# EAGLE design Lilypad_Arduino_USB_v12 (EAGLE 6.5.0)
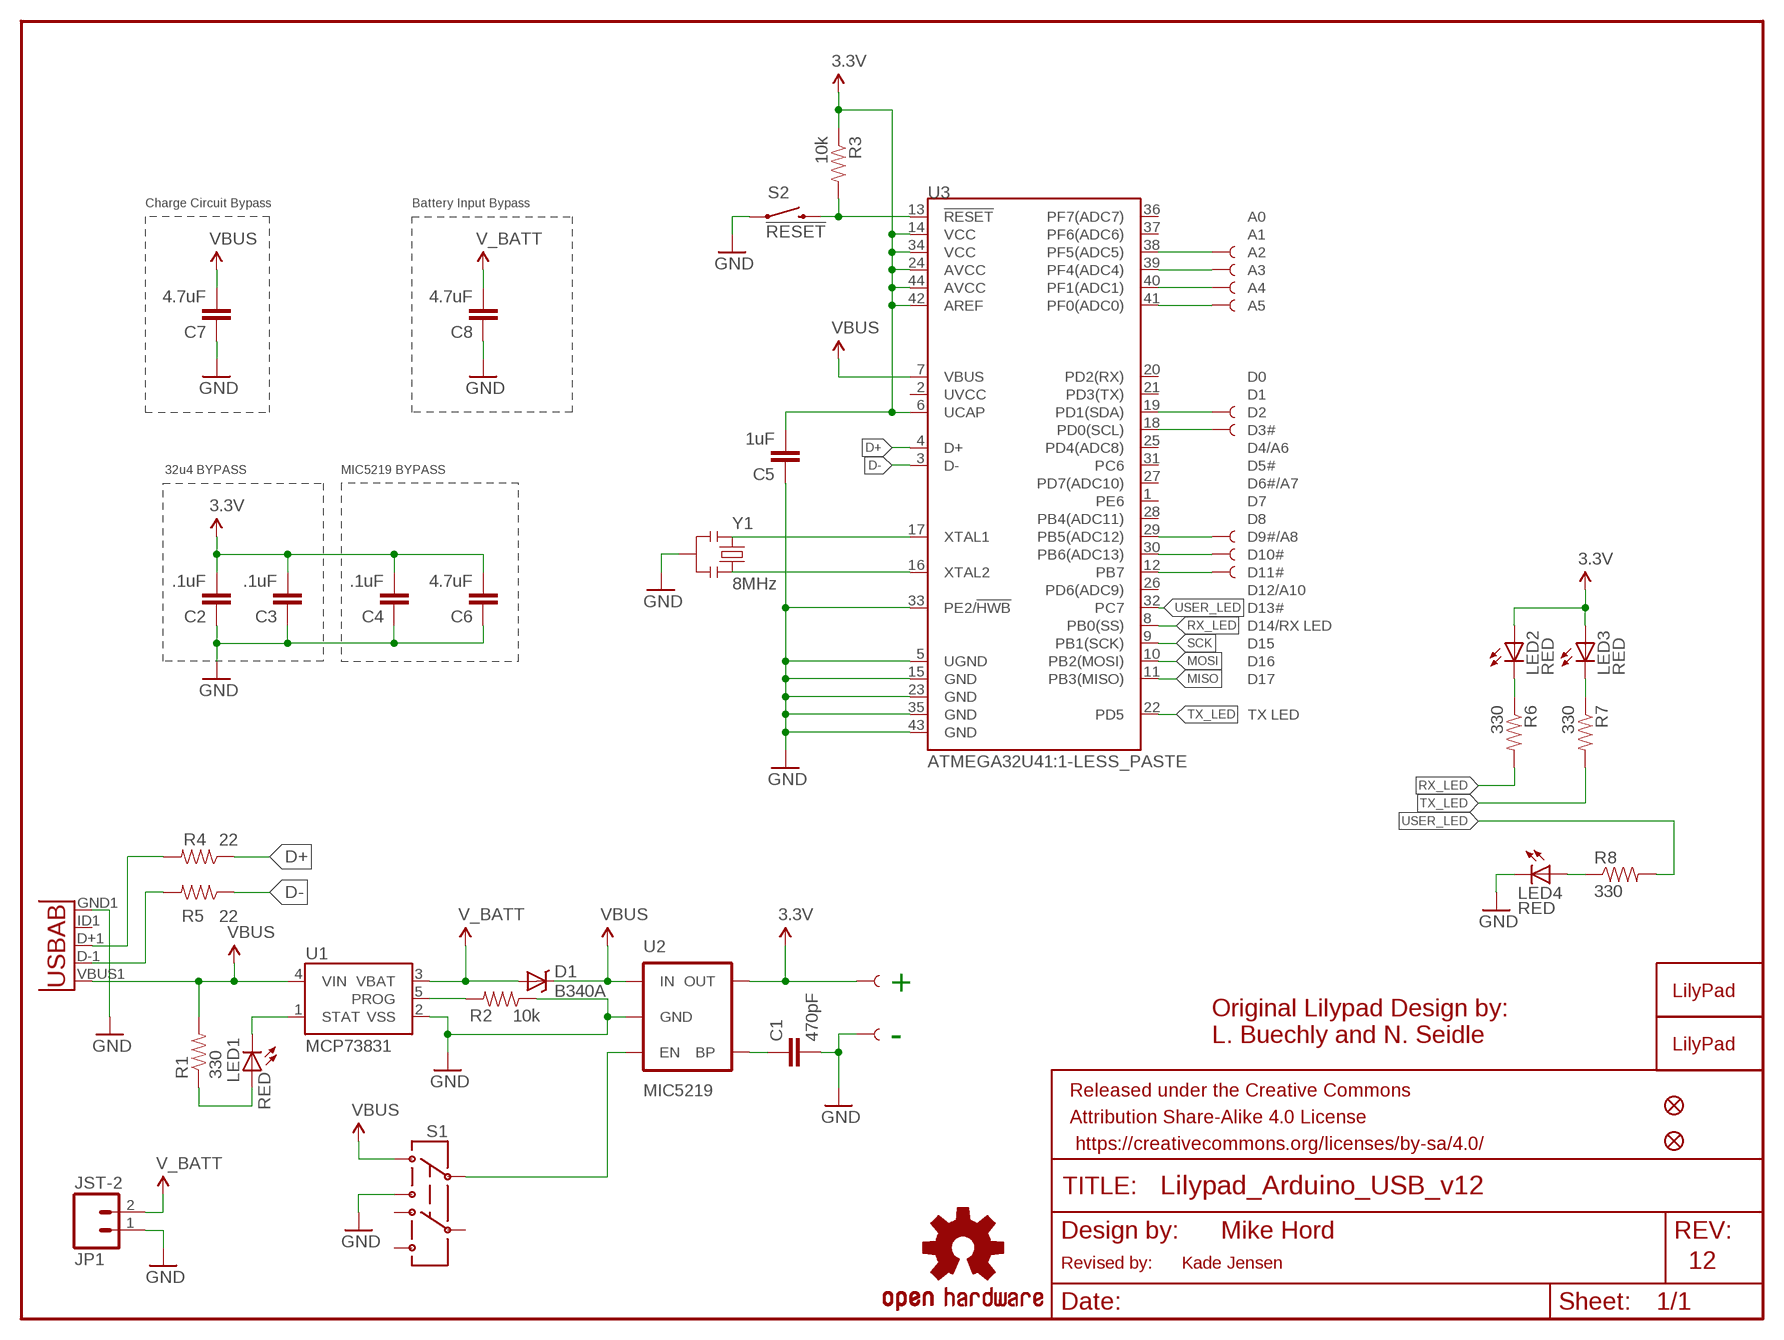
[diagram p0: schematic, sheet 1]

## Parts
+  SEWTAP9  [PETAL-LONG-1-2SIDE]
-  SEWTAP9  [PETAL-LONG-1-2SIDE]
A2  SEWTAP9  [PETAL-LONG-1-2SIDE]
A3  SEWTAP9  [PETAL-LONG-1-2SIDE]
A4  SEWTAP9  [PETAL-LONG-1-2SIDE]
A5  SEWTAP9  [PETAL-LONG-1-2SIDE]
C1  470pF  CAP0603-CAP  [0603-CAP]
C2  .1uF  CAP0603-CAP  [0603-CAP]
C3  .1uF  CAP0603-CAP  [0603-CAP]
C4  .1uF  CAP0603-CAP  [0603-CAP]
C5  1uF  CAP0603-CAP  [0603-CAP]
C6  4.7uF  CAP0603-CAP  [0603-CAP]
C7  4.7uF  CAP1206  [1206]
C8  4.7uF  CAP1206  [1206]
D1  B340A  DIODE-SCHOTTKY-B340A  [SMA-DIODE]
D5  SEWTAP9  [PETAL-LONG-1-2SIDE]
D6  SEWTAP9  [PETAL-LONG-1-2SIDE]
D9  SEWTAP9  [PETAL-LONG-1-2SIDE]
D10  SEWTAP9  [PETAL-LONG-1-2SIDE]
D11  SEWTAP9  [PETAL-LONG-1-2SIDE]
FRAME1  FRAME-LETTER  [CREATIVE_COMMONS]
JP1  JST-2  M02-JST-2MM-SMT  [JST-2-SMD]
JP2  FIDUCIAL1X2  [FIDUCIAL-1X2]
JP3  FIDUCIAL1X2  [FIDUCIAL-1X2]
LED1  RED  LED0603  [LED-0603]
LED2  RED  LED0603  [LED-0603]
LED3  RED  LED0603  [LED-0603]
LED4  RED  LED0603  [LED-0603]
R1  330  RESISTOR0603-RES  [0603-RES]
R2  10k  RESISTOR0603-RES  [0603-RES]
R3  10k  RESISTOR0603-RES  [0603-RES]
R4  22  RESISTOR0603-RES  [0603-RES]
R5  22  RESISTOR0603-RES  [0603-RES]
R6  330  RESISTOR0603-RES  [0603-RES]
R7  330  RESISTOR0603-RES  [0603-RES]
R8  330  RESISTOR0603-RES  [0603-RES]
S1  SWITCH-DPDTAYZ0202  [AYZ0202]
S2  !RESET  SWITCH-MOMENTARY-2SMD  [TACTILE_SWITCH_SMD]
U1  MCP73831  [SOT23-5]
U2  MIC5219  V_REG_MIC52193.3V  [SOT23-5]
U3  ATMEGA32U41:1-LESS_PASTE  [QFN-44-NOPAD_1:1-LESS_PASTE]
U5  USB-ABCONN-11794  [USB-AB-MICRO-SMD_V03]
U$1  LOGO-LPLPA  [LOGO-LPA]
U$5  OSHW-LOGOM  [OSHW-LOGO-M]
U$13  LOGO-LPLP  [LOGO-LILYPAD]
Y1  8MHz  RESONATOR8MHZ  [RESONATOR-SMD]

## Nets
3.3V: +.1 C2.2 C3.2 C4.2 C5.2 C6.2 LED2.A LED3.A R3.1 U2.5(OUT) U3.6(UCAP) U3.14(VCC) U3.24(AVCC) U3.34(VCC) U3.42(AREF) U3.44(AVCC)
5V: C7.2 D1.C R1.2 S1.1 U1.4(VIN) U2.1(IN) U3.7(VBUS) U5.VBUS1(VBUS) ; supply symbol labelled VBUS
D+: R4.1 U3.4(D+)
D-: R5.1 U3.3(D-)
GND: -.1 C1.2 C2.1 C3.1 C4.1 C5.1 C6.1 C7.1 C8.1 JP1.1 LED4.C R2.1 S1.3 S2.1 U1.2(VSS) U2.2(GND) U3.5(UGND) U3.15(GND) U3.23(GND) U3.33(PE2/!HWB) U3.35(GND) U3.43(GND) U5.GND1(GND) Y1.2
MISO: U3.11(PB3(MISO))
MOSI: U3.10(PB2(MOSI))
N$1: LED2.C R6.1
N$2: S1.2 U2.3(EN)
N$3: LED1.A R1.1
N$4: LED1.C U1.1(STAT)
N$5: U3.17(XTAL1) Y1.1
N$6: R2.2 U1.5(PROG)
N$7: U3.16(XTAL2) Y1.3
N$8: C1.1 U2.4(BP)
N$9: D11.1 U3.12(PB7)
N$10: D10.1 U3.30(PB6(ADC13))
N$11: D9.1 U3.29(PB5(ADC12))
N$12: D5.1 U3.19(PD1(SDA))
N$13: D6.1 U3.18(PD0(SCL))
N$14: A5.1 U3.41(PF0(ADC0))
N$15: A4.1 U3.40(PF1(ADC1))
N$16: A3.1 U3.39(PF4(ADC4))
N$17: A2.1 U3.38(PF5(ADC5))
N$18: LED4.A R8.1
N$19: R5.2 U5.D-1(D-)
N$20: R4.2 U5.D+1(D+)
N$21: LED3.C R7.1
RESET: R3.2 S2.3 U3.13(!RESET)
RX_LED: R6.2 U3.8(PB0(SS))
SCK: U3.9(PB1(SCK))
TX_LED: R7.2 U3.22(PD5)
USER_LED: R8.2 U3.32(PC7)
V_BATT: C8.2 D1.A JP1.2 U1.3(VBAT)
Unconnected: S1.4 S1.5 S1.6 U3.1(PE6) U3.2(UVCC) U3.20(PD2(RX)) U3.21(PD3(TX)) U3.25(PD4(ADC8)) U3.26(PD6(ADC9)) U3.27(PD7(ADC10)) U3.28(PB4(ADC11)) U3.31(PC6) U3.36(PF7(ADC7)) U3.37(PF6(ADC6)) U5.ID1(USBID)

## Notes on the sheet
- Charge Circuit Bypass | Battery Input Bypass
- 32u4 BYPASS | MIC5219 BYPASS
- +
- Original Lilypad Design by:
- - | L. Buechly and N. Seidle
- Mike Hord
- Revised by: | Kade Jensen | 12

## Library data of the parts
+ - A2-A5 D5 D6 D9-D11 = LilyPad-Wearables:SEWTAP; NO_PART: 1
C1 = SparkFun-Passives:CAP: Capacitor; PROD_ID: CAP-07884
C2-C4 = SparkFun-Passives:CAP: Capacitor; PROD_ID: CAP-00810
C5 = SparkFun-Passives:CAP: Capacitor; PROD_ID: CAP-00868
C6 = SparkFun-Passives:CAP: Capacitor; PROD_ID: CAP-08280
C7 C8 = SparkFun-Passives:CAP: Capacitor; PROD_ID: CAP-10300
D1 = SparkFun-DiscreteSemi:DIODE-SCHOTTKY: Schottky diodes in SFE's production catalog; PROD_ID: DIO-09886
FRAME1 = SparkFun-Aesthetics:FRAME-LETTER: Schematic Frame
JP1 = SparkFun-Connectors:M02: Standard 2-pin 0.1" header. Use with; PROD_ID: CONN-08352
JP2 JP3 = SparkFun:FIDUCIAL: Fiducial Alignment Points
LED1-LED4 = SparkFun-LED:LED: LEDs; PROD_ID: DIO-00819
R1 R7 R8 = SparkFun-Passives:RESISTOR: Resistor; PROD_ID: RES-00818
R2 R3 = SparkFun-Resistors:RESISTOR: Resistor; PROD_ID: RES-00824
R4 R5 = SparkFun-Resistors:RESISTOR: Resistor; PROD_ID: RES-08698
R6 = SparkFun-Resistors:RESISTOR: Resistor; PROD_ID: RES-00818
S1 = SparkFun-Electromechanical:SWITCH-DPDT: DPDT Version of the COM-00597; PROD_ID: SWCH-08179; VALUE: DPDT
S2 = SparkFun-Electromechanical:SWITCH-MOMENTARY-2: Various NO switches- pushbuttons, reed, etc; PROD_ID: SWCH-08247
U1 = SparkFun-PowerIC:MCP73831: Miniature single cell, fully integrated Li-Ion, Li-polymer charge management controller http://ww1.microchip.com/downloads/en/DeviceDoc/21984a.pdf IC-09995; PROD_ID: IC-09995
U2 = SparkFun-PowerIC:V_REG_MIC5219: V_REG MIC5219 Standard 3.3V and 5V 500mA LDO voltage regulator in SOT-23 layout. Micrel part MIC5219. BP (by-pass) pin is used to lower output noise with 470pF cap, may be left open.; PROD_ID: VREG-09872; VALUE: MIC5219 3.3V
U3 = Testing:ATMEGA32U4: Atmel 44-pin 8-bit Microcontroller with 32KBytes of ISP Flash and USB Controller; PROD_ID: IC-10828
U5 = SparkFun-Connectors:USB-AB: This is a USB AB connector that is compatible with USB OTG. i.e. this connector can serve as a host or device; PROD_ID: CONN-11794
U$1 = LilyPad-Wearables:LOGO-LP
U$5 = SparkFun:OSHW-LOGO: Open Source Hardware Logo This logo indicates the piece of hardware it is found on incorporates a OSHW license and/or adheres to the definition of open source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
U$13 = LilyPad-Wearables:LOGO-LP; NO_PART: 1
Y1 = SparkFun-FreqCtrl:RESONATOR: Resonator Small SMD resonator. Used, eg, on the Arduino Pro/ Pro Mini boards. 8MHz- XTAL-08895 16MHz- XTAL-08900; PROD_ID: XTAL-08895; VALUE: 8MHZ

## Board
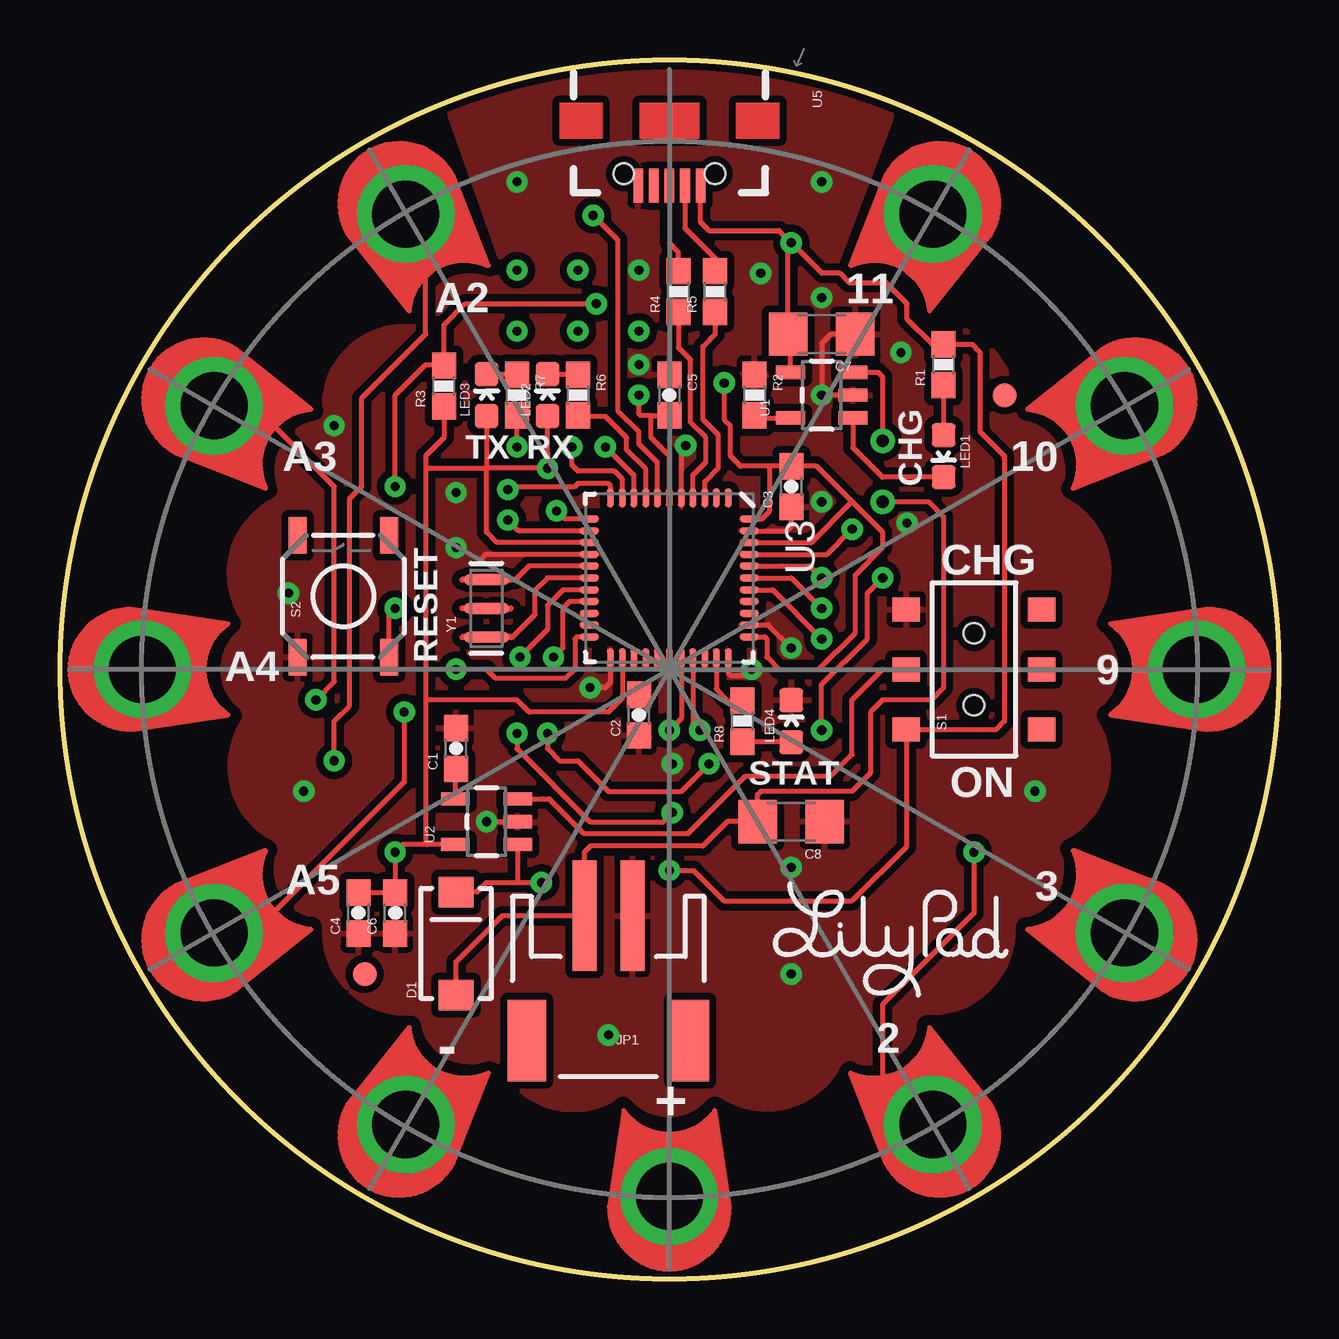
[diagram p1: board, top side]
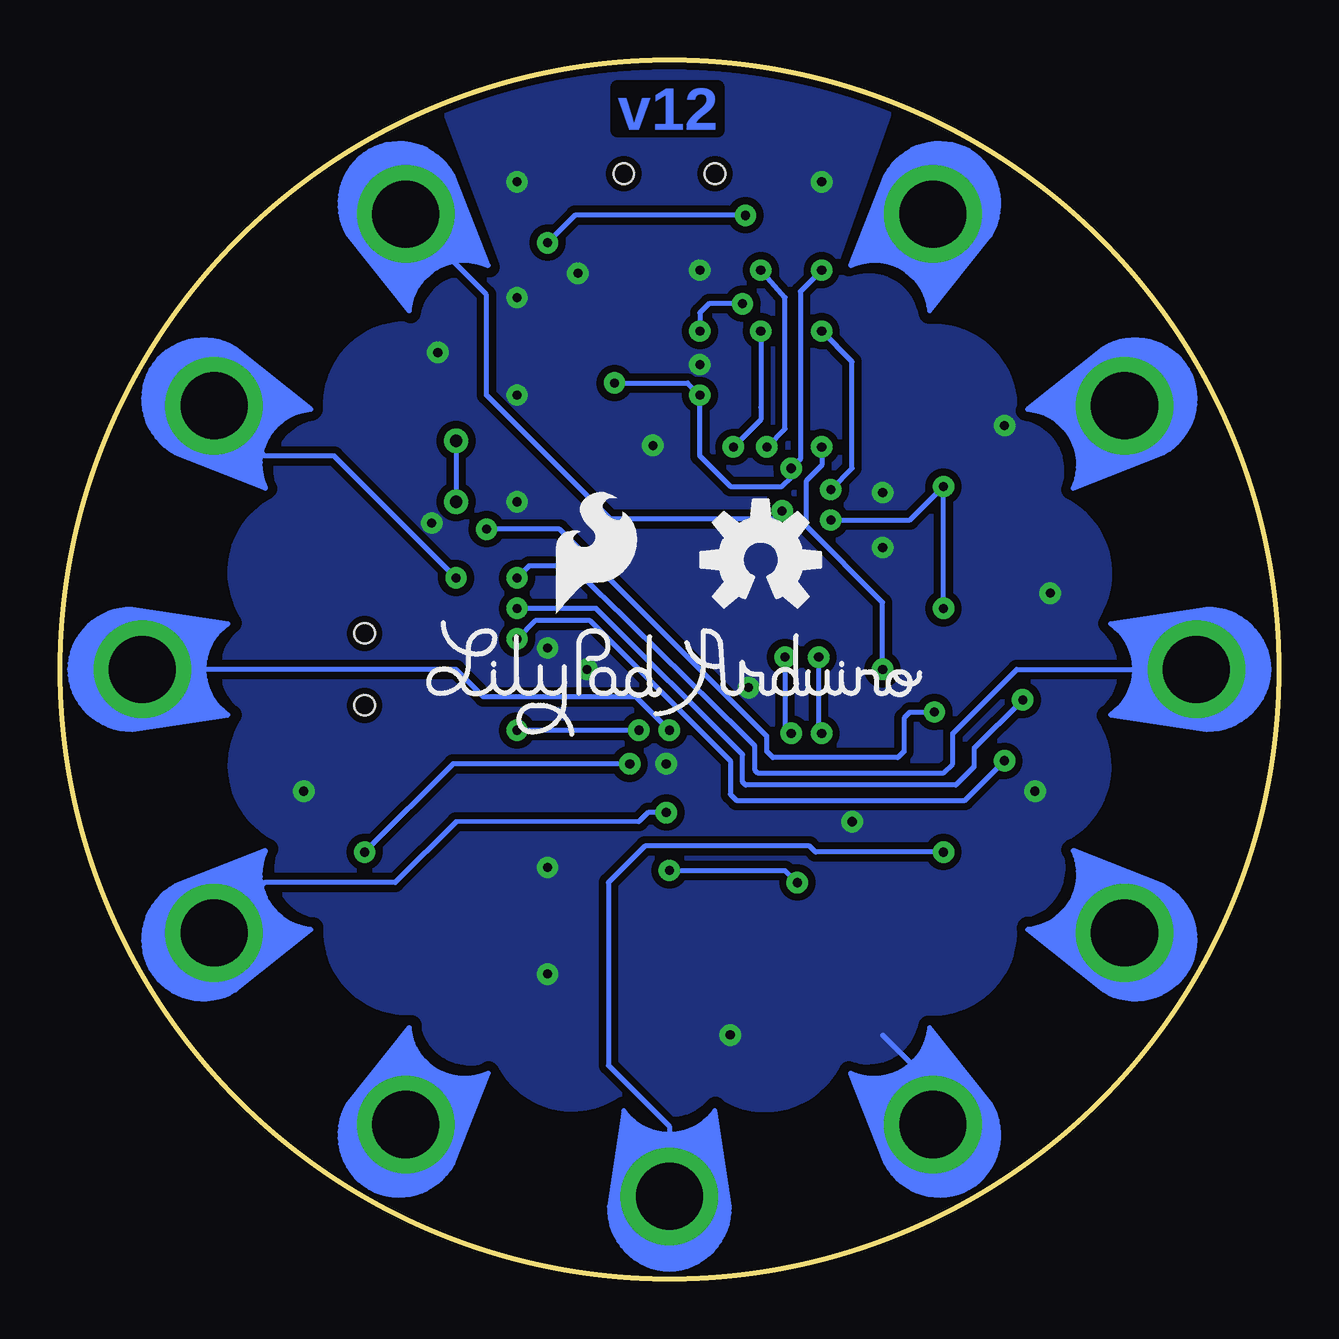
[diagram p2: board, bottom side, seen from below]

Size 50.8 x 50.8 mm. Coordinates in mm from the lower left corner, seen from the top.
Outline: circle at 25.4,25.4 radius 25.4
Copper layers (1*16): Top 0.035mm / dielectric 1.5mm / Bottom 0.035mm
Design rules "SparkFun-2-layer": minimum track width 7mil, minimum drill 15mil, track to track 8mil, track to pad 8mil, pad to pad 8mil, via to via 8mil, smd to smd 8mil, copper to edge 8mil, drill to drill 8mil, minimum pad ring 12mil, minimum via ring 10mil, stop-mask expansion 4mil, vias tented up to drill 20mil, thermal gap 10mil
tRestrict: area 2.1,32.9 to 10.5,40.7; area 40.3,10.1 to 48.7,17.9; area 0.3,22.4 to 7.1,28.6; area 43.7,22.2 to 50.5,28.4; area 32.9,2 to 40.6,10.5; area 40.3,32.9 to 48.8,40.6; area 2,10.2 to 10.5,17.9; area 10.2,40.3 to 17.9,48.8; area 32.9,40.3 to 40.7,48.7; area 10.1,2.1 to 17.9,10.5; area 0.3,27.3 to 8.6,35.3; area 5.2,36.2 to 14.6,45.6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
bRestrict: area 0.3,22.4 to 7.1,28.6; area 43.7,22.2 to 50.5,28.4; area 32.9,2 to 40.6,10.5; area 40.3,32.9 to 48.8,40.6; area 2,10.2 to 10.5,17.9; area 10.2,40.3 to 17.9,48.8; area 32.9,40.3 to 40.7,48.7; area 10.1,2.1 to 17.9,10.5; area 0.3,27.3 to 8.6,35.3; area 5.2,36.2 to 14.6,45.6; area 42.2,27.3 to 50.5,35.3; area 36.2,36.2 to 45.6,45.6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

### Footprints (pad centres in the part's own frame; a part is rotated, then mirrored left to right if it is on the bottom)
PETAL-LONG-1-2SIDE = drill 2.794 pad 4.064: 1 0.03,0
0603-CAP = smd 1.1 x 1: 1 -0.85,0; 2 0.85,0
1206 = smd 1.6 x 1.8: 1 -1.4,0; 2 1.4,0
SMA-DIODE = smd 1.27 x 1.47: A -2.15,0; C 2.15,0
JST-2-SMD = smd 1 x 4.6: 1 -1,-3.7; 2 1,-3.7 | smd 1.6 x 3.4: NC1 -3.4,1.5; NC2 3.4,1.5
FIDUCIAL-1X2 = smd 1 x 1: 1 0,0
LED-0603 = smd 1 x 1: A 0,-0.877; C 0,0.877
0603-RES = smd 1.1 x 1: 1 -0.85,0; 2 0.85,0
AYZ0202 = smd 1 x 1.15: 1 -2.5,2.825; 2 0,2.825; 3 2.5,2.825; 4 -2.5,-2.825; 5 0,-2.825; 6 2.5,-2.825 | hole 0.85: 1.5,0; -1.5,0
TACTILE_SWITCH_SMD = smd 1.524 x 0.762: 1 -2.54,1.905; 2 2.54,1.905; 3 -2.54,-1.905; 4 2.54,-1.905
SOT23-5 = smd 0.55 x 1.2: 1 -0.95,-1.3; 2 0,-1.3; 3 0.95,-1.3; 4 0.95,1.3; 5 -0.95,1.3
QFN-44-NOPAD_1:1-LESS_PASTE = smd 0.8 x 0.3: 1 -3.337,2.458; 2 -3.337,1.958; 3 -3.337,1.479; 4 -3.337,0.979; 5 -3.337,0.5; 6 -3.337,0; 7 -3.337,-0.5; 8 -3.337,-0.979; 9 -3.337,-1.479; 10 -3.337,-1.958; 11 -3.337,-2.458; 23 3.337,-2.458; 24 3.337,-1.958; 25 3.337,-1.479; 26 3.337,-0.979; 27 3.337,-0.5; 28 3.337,0; 29 3.337,0.5; 30 3.337,0.979; 31 3.337,1.479; 32 3.337,1.958; 33 3.337,2.458 | smd 0.3 x 0.8: 12 -2.458,-3.337; 13 -1.958,-3.337; 14 -1.479,-3.337; 15 -0.979,-3.337; 16 -0.5,-3.337; 17 0,-3.337; 18 0.5,-3.337; 19 0.979,-3.337; 20 1.479,-3.337; 21 1.958,-3.337; 22 2.458,-3.337; 34 2.458,3.337; 35 1.958,3.337; 36 1.479,3.337; 37 0.979,3.337; 38 0.5,3.337; 39 0,3.337; 40 -0.5,3.337; 41 -0.979,3.337; 42 -1.479,3.337; 43 -1.958,3.337; 44 -2.458,3.337
USB-AB-MICRO-SMD_V03 = smd 1.4 x 0.4: D+1 2.7,0; D-1 2.7,0.65; GND1 2.7,-1.3; ID1 2.7,-0.65; VBUS1 2.7,1.3 | hole 0.85: 2.2,1.9; 2.2,-1.9
RESONATOR-SMD = smd 0.45 x 1.905: 1 -1.2,0; 2 0,0; 3 1.2,0

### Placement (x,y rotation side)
+  25.4,3.4 90 top
-  14.4,6.4 60 top
A2  14.4,44.4 300 top
A3  6.4,36.4 330 top
A4  3.4,25.4 0 top
A5  6.4,14.4 30 top
C1  16.51,22.1 90 top
C2  24.13,23.5 90 top
C3  30.48,33.02 90 top
C4  12.45,15.24 90 top
C5  25.4,36.83 270 top
C6  13.97,15.24 90 top
C7  31.75,39.37 180 top
C8  30.48,19.05 180 top
D1  16.51,13.97 90 top
D5  36.4,6.4 120 top
D6  44.4,14.4 150 top
D9  47.4,25.4 180 top
D10  44.4,36.4 210 top
D11  36.4,44.4 240 top
FRAME1  not placed on the board
JP1  22.86,11.43 180 top
JP2  12.7,12.7 0 top
JP3  39.37,36.83 0 top
LED1  36.83,34.29 180 top
LED2  20.32,36.83 0 top
LED3  17.78,36.83 0 top
LED4  30.48,23.24 0 top
R1  36.83,38.1 90 top
R2  28.96,36.83 270 top
R3  16,37.21 90 top
R4  25.78,41.15 90 top
R5  27.3,41.15 90 top
R6  21.59,36.83 270 top
R7  19.05,36.83 270 top
R8  28.45,23.24 90 top
S1  38.1,25.4 90 top
S2  11.81,28.45 90 top
U1  31.75,36.83 90 top
U2  17.78,19.05 90 top
U3  25.4,29.21 270 top
U5  25.4,48.26 270 top
U$1  25.4,25.4 0 bottom
U$5  21.59,29.97 0 bottom
U$7  [SFE_LOGO_FLAME_.2]  30.48,27.43 0 bottom
U$13  34.67,14.48 0 top
Y1  17.78,27.94 90 top

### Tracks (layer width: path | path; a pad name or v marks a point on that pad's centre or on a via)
3.3V  (via drill 0.38)
  Top 0.203: 16.19,18.1 U2.5 15.3,18.1 | LED2.A 20.32,34.42 v20.32,33.78 17.78,33.78 | 15.3,18.1 15.24,18.16 15.24,24.13 | 15.3,18.1 14.29,18.1 v13.97,17.78 C6.2 C4.2 | R3.1 16,35.05 15.24,34.29 15.24,33.78 | 29.59,33.87 C3.2 31.53,33.87 33.02,32.38 | U3.44 29.25,31.67 29.59,32 29.59,33.87 | 15.24,24.13 19.05,24.13 19.56,23.62 22.86,23.62 23.44,24.2 23.44,24.34 | U3.24 23.44,24.34 | C2.2 23.44,24.34 | 24.64,35.98 24.22,35.98 24.13,36.07 v24.13,36.83 | U3.6 25.4,34.29 24.64,35.05 24.64,35.98 | 24.64,35.98 C5.2 | v27.69,37.34 27.69,35.81 27.94,35.56 27.94,34.29 28.36,33.87 29.59,33.87 | U3.34 29.38,26.75 29.46,26.67 29.46,25.91 29.97,25.4 31.62,25.4 33.15,26.92 33.15,29.34 34.29,30.48 34.29,31.11 33.02,32.38 | U3.42 31.32,30.69 33.02,32.38 | U3.14 18.21,30.69 17.78,31.11 17.78,33.78 | 15.24,33.78 17.78,33.78 | 17.78,33.78 | 17.78,33.78 | LED3.A 17.78,33.78 | 17.78,33.78 | 15.24,33.78 | 15.24,33.78 15.24,24.13
  Bottom 0.203: v19.05,42.04 19.94,41.15 19.94,34.16 v20.32,33.78 | v13.97,17.78 19.3,17.78 19.56,18.03 26.42,18.03 27.94,16.51 27.94,8.89 25.4,6.35 +.1 | v20.32,33.78 | v20.32,33.78 20.32,33.4 20.7,33.02 22.86,33.02 24.13,34.29 v24.13,36.83 24.64,37.34 v27.69,37.34
5V  (via drill 0.38)
  Top 0.203: U3.7 24.9,34.03 24.13,34.8 24.13,35.31 23.24,36.2 23.24,43.31 v22.22,44.32 | v25.4,17.02 26.42,17.02 27.69,15.75 33.02,15.75 35.27,18 S1.1 39.03,22.9 39.37,23.24 39.37,34.29 38.35,35.31 38.35,38.61 38.01,38.95 R1.2 36.36,38.95 35.31,40 35.31,40.64 34.42,41.53 32.89,41.53 32.51,41.91 31.75,41.91 v30.48,43.18 | v30.48,43.18 29.97,43.69 27.05,43.69 26.7,44.04 U5.VBUS1 | v30.48,43.18 30.35,43.05 C7.2 30.45,39.27 U1.4 | 19.05,16.51 17.78,16.51 17.39,16.12 D1.C | 19.05,16.51 v20.07,16.51 | v20.07,16.51 | U2.1 19.08,16.54 19.05,16.51 | D1.C | U5.VBUS1
  Bottom 0.203: v22.22,44.32 29.34,44.32 v30.48,43.18 | v25.4,17.02 20.57,17.02 v20.07,16.51
D+
  Top 0.203: R4.1 25.78,38.81 26.29,38.3 26.29,35.69 26.92,35.05 26.92,34.04 26.38,33.49 U3.4
D-
  Top 0.203: R5.1 27.3,39.37 26.8,38.86 26.8,35.81 27.43,35.18 27.43,33.78 26.88,33.23 U3.3
GND  (via drill 0.38)
  Top 0.203: U1.2 v31.75,36.83 31.75,38.99 32.13,39.37 C7.1 | U2.2 v17.78,19.05 | C3.1 30.48,31.37 30.28,31.17 U3.43 | U3.15 17.74,30.19 17.65,30.1 | U3.23 22.94,24.85 22.73,24.64 v22.1,24.64 | U3.5 25.9,34.55 v26.09,34.73 | U3.33 27.86,25.23 27.94,25.15 28.57,25.15 v28.83,25.4 | U3.35 29.52,27.25 v30.48,26.29
  Bottom 0.203: -.1 14.41,8.06 16.51,10.16
  other vias: 24.13,42.04 22.86,10.16 30.48,12.7 10.16,20.32 29.21,41.91 9.53,28.57 24.13,38.1 31.75,40.89 19.05,45.72 16.51,30.48 16.51,32.77 35.31,31.5 31.75,32.38 25.53,21.46 30.48,17.14 35.05,38.61 11.43,35.56 31.75,45.72 40.64,20.32
  pour Top (isolate 0.305): 50.8,25.4 arc90 25.4,50.8 arc90 0,25.4 arc90 25.4,0 arc90
  pour Bottom (isolate 0.305): 50.8,25.4 arc90 25.4,50.8 arc90 0,25.4 arc90 25.4,0 arc90
MISO  (via drill 0.38)
  Top 0.203: v18.67,32.89 18.8,33.02 21.46,33.02 21.59,33.15 22.86,33.15 22.94,33.06 U3.11
  Bottom 0.203: 17.78,33.78 17.78,38.23 v19.05,39.5 | 17.78,33.78 | 17.78,33.78 v18.67,32.89
MOSI  (via drill 0.38)
  Top 0.203: U3.10 23.44,33.33 23.11,33.66 21.59,33.66 21.34,33.91 v21.34,34.67
  Bottom 0.203: v21.59,42.04 20.57,40.89 20.57,35.43 v21.34,34.67
N$1
  Top 0.203: LED2.C 21.56,37.71 R6.1
N$2
  Top 0.203: U2.3 20.13,20 20.39,20 21.84,18.54 26.16,18.54 28.57,20.95 32.13,20.95 33.02,21.84 33.02,24.13 34.29,25.4 S1.2
N$3
  Top 0.203: R1.1 LED1.A
N$4
  Top 0.203: U1.1 33.05,34.64 34.28,33.41 LED1.C
N$5
  Top 0.203: Y1.1 18.87,26.74 19.81,27.69 19.81,28.7 20.32,29.21 | U3.17 20.32,29.21 | 20.32,29.21
N$6
  Top 0.203: R2.2 arc90 29.06,35.88 U1.5
N$7
  Top 0.203: Y1.3 18.98,29.14 19.55,29.71 U3.16
N$8
  Top 0.203: U2.4 16.48,21.22
  Top 0.254: 16.48,21.22 C1.1
N$9  (via drill 0.38)
  Top 0.203: U3.12 21.04,31.67 v20.7,32
  Bottom 0.203: v20.7,32 21.04,31.67 27.86,31.67 33.02,36.83 33.02,41.01 D11.1
N$10  (via drill 0.38)
  Top 0.203: v31.75,22.86 31.75,24.76 33.66,26.67 33.66,28.57 v34.29,29.21 | U3.30 26.38,23.15 v26.67,22.86
  Bottom 0.203: v26.67,22.86 v31.75,22.86 | v34.29,29.21 39.37,34.29 42.28,34.29 D10.1
N$11  (via drill 0.38)
  Top 0.203: U3.29 25.9,23.36 v25.4,22.86
  Bottom 0.203: v25.4,22.86 26.8,24.26 33.15,24.26 34.29,25.4 D9.1
N$12  (via drill 0.38)
  Top 0.203: v20.32,22.73 20.32,22.1 20.83,21.59 21.59,21.59 22.86,20.32 25.91,20.32 v27.05,21.46 | v38.1,17.78 38.1,15.24 34.29,11.43 34.29,8.52 D5.1 | U3.19 21.25,28.23 20.95,27.94 20.95,26.29 v20.57,25.91
  Bottom 0.203: v27.05,21.46 34.42,21.46 v38.1,17.78 | v20.57,25.91 20.57,22.99 v20.32,22.73
N$13  (via drill 0.38)
  Top 0.203: v19.05,22.73 19.05,22.1 22.1,19.05 25.15,19.05 v25.53,19.43 | U3.18 20.96,28.71 20.32,28.07 20.32,27.05 v19.18,25.91
  Bottom 0.203: D6.1 42.28,16.51 36.83,16.51 34.29,19.05 26.67,19.05 26.29,19.43 v25.53,19.43 | v19.18,25.91 19.18,22.86 v19.05,22.73
N$14  (via drill 0.38)
  Top 0.203: v14.35,23.62 14.35,20.7 7.62,13.97 6.87,13.97 A5.1 | U3.41 31.97,30.19 v33.02,31.24
  Bottom 0.203: v14.35,23.62 15.37,23.62 15.62,23.37 15.62,21.97 15.87,21.72 21.08,21.72 21.34,21.97 21.34,22.61 29.97,31.24 v33.02,31.24
N$15  (via drill 0.38)
  Top 0.203: U3.40 30.11,29.71 31.25,29.71 v31.75,29.21
  Bottom 0.203: A4.1 10.92,25.4 13.59,22.73 13.59,21.46 13.97,21.08 21.72,21.08 21.84,21.21 21.84,22.22 22.35,22.73 28.19,28.45 28.2,28.45 29.46,29.71 31.25,29.71 v31.75,29.21
N$16  (via drill 0.38)
  Top 0.203: v10.67,24.13 11.43,24.89 11.43,33.02 8.06,36.38 A3.1 | U3.39 30.48,29.21 v31.75,27.94
  Bottom 0.203: v10.67,24.13 12.7,22.1 12.7,21.34 13.46,20.57 22.22,20.57 22.35,20.7 22.35,21.84 28.45,27.94 v31.75,27.94
N$17  (via drill 0.38)
  Top 0.203: U3.38 29.71,28.71 v31.75,26.67 | v11.43,21.59 11.43,23.24 12.06,23.88 12.06,32.51 12.57,33.02 12.57,36.7 15.24,39.37 15.24,43.55 A2.1 14.35,44.31
  Bottom 0.203: v11.43,21.59 13.08,19.94 22.61,19.94 22.86,20.19 22.86,21.59 28.7,27.43 30.99,27.43 v31.75,26.67
N$18
  Top 0.203: R8.1 30.45,22.39 LED4.A
N$19
  Top 0.203: R5.2 27.3,42.55 26.05,43.8 U5.D-1 | U5.D-1
N$20
  Top 0.203: R4.2 25.78,42.8 25.4,43.18 U5.D+1
N$21
  Top 0.203: LED3.C 19.02,37.71 R7.1
RESET  (via drill 0.38)
  Top 0.203: v18.67,31.62 19.08,31.21 19.12,31.17 U3.13 | v22.35,40.64 16.89,40.64 16,39.75 R3.2 15.96,38.1 15.24,38.1 13.97,36.83 v13.97,33.02 | S2.3 13.72,27.69 v13.97,27.94
  Bottom 0.203: v22.35,40.64 23.75,40.64 24.13,40.26 v24.13,39.5 | v18.67,31.62 15.37,31.62 v13.97,33.02 | v13.97,27.94 v13.97,33.02 | v13.97,33.02
RX_LED
  Top 0.203: U3.8 24.42,33.74 23.62,34.54 23.62,35.05 22.73,35.94 21.63,35.94 R6.2
SCK  (via drill 0.38)
  Top 0.203: U3.9 23.92,33.48 v22.73,34.67
  Bottom 0.203: v21.59,39.5 21.59,36.32 21.59,35.81 v22.73,34.67
TX_LED  (via drill 0.38)
  Top 0.203: v19.05,34.67 R7.2 | v16.51,25.4 17.78,25.4 18.16,25.02 21.08,25.02 21.46,25.4 21.46,26.67 21.54,26.75 U3.22
  Bottom 0.203: v19.05,34.67 19.05,33.91 19.68,33.27 19.68,31.37 16.51,28.19 v16.51,25.4
USER_LED
  Top 0.203: R8.2 27.85,24.09 27.4,24.54 27.36,24.58 U3.32
V_BATT  (via drill 0.51)
  Top 0.203: U1.3 34.1,37.78 34.29,37.59 v34.29,34.92 | v34.29,32.38 36.2,32.38 36.83,31.75 36.83,24.64 36.32,24.13 34.29,24.13 33.78,23.62 33.78,21.08 33.02,20.32 29.21,20.32 29.08,20.19 C8.2 27.81,19.05 26.8,18.03 22.11,18.03 21.86,17.78 JP1.2 18.43,15.13 16.51,13.21 D1.A
  Bottom 0.203: v34.29,34.92 v34.29,32.38

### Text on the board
Bottom: v12
tPlace: A2 | 11 | TX | RX | A3 | CHG | 10 | RESET | CHG | A4 | 9 | STAT | ON | A5 | 3 | 2 | - | +
tDocu: Mike Hord | Revised by: Kade Jensen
